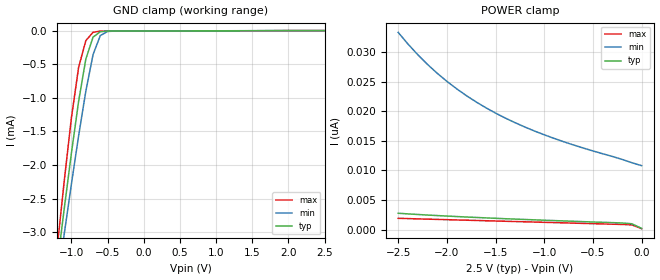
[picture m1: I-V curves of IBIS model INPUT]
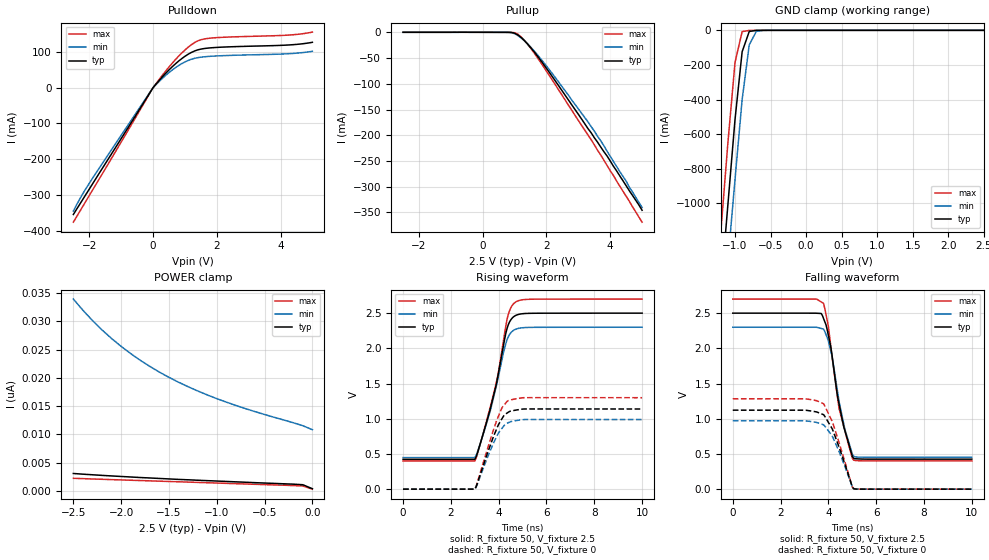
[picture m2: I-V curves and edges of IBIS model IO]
|   PERICOM SEMICONDUCTOR CORP
|   IBIS Model of PI4ULS3V204
|   Product Family: ULS
|   TSSOP-14 (L) Package
[IBIS Ver] 3.2
[Comment char] |_char
[File Name] pi4uls3v204_l_25v.ibs
[File Rev] 1.0
[Source] File originated at Pericom Semiconductor Corp.
[Date] 09/06/2017
[Disclaimer] (C) Copyright PERICOM Semiconductor Corporation
   All rights reserved
  Pericom Semiconductor Corporation hereby grants the user of
  this IBIS model a non-exclusive, nontransferable license to
  use this IBIS model under the following terms.
  This IBIS model is provided on an "AS IS" basis and Pericom
  makes absolutely no warranty with respect to the information
  contained herein. PERICOM DISCLAIMS AND CUSTOMER WAIVES ALL
  WARRANTIES, EXPRESSED OR IMPLIED, INCLUDING WARRANTIES OF
  MERCHANTABILITY OR FITNESS FOR A PARTICULAR PURPOSE. The
  entire risk as to quality and performance is with the customer.
  Accordingly, in no event shall the company be liable for any
  damages, whether in contract or tort, including any lost
  profits or other incidental, consequential, exemplary, or
  punitive damages arising out of the use or application of the
  IBIS model provided in this package. Further, Pericom reserves
  the right to make changes without notice to any product herein
  to improve reliability, function, or design. Pericom does not
  convey any license under patent rights or any other intellectual
  property rights, including those of third parties.
  The user is granted this license only to use the IBIS model
  and is not granted rights to sell, load, rent, lease or license
  the IBIS model in whole or in part, or in modified form to anyone
  other than user. User may modify the IBIS model to suit its specific
  application but rights to derivative works and such modifications
  shall belong to Pericom.
  Pericom is not obligated to provide maintenance or support
  for the licensed IBIS model.
  Contact Pericom at ATTN: APPLICATION ENGINEERING / IBIS MODELS
  1545 Barber Lane Milpitas, CA 95035 USA.
[Component] PI4ULS3V204
[Manufacturer] Pericom Semiconductor Corp.
[Package]
| variable   typ   min   max
R_pkg   0.04200   0.03995   0.04405
L_pkg   2.30669n   2.21200n   2.40138n
C_pkg   0.21108p   0.20715p   0.21500p
[Pin] signal_name  model_name   R_pin   L_pin   C_pin
1   VCCA   POWER   0.03604  2.91900n  0.20300p
2   A1   IO   0.03631  2.73467n  0.19100p
3   A2   IO   0.03658  2.55033n  0.17900p
4   A3   IO   0.03686  2.36600n  0.16700p
5   A4   IO   0.03658  2.55033n  0.17900p
6   NC   NC   0.03631  2.73467n  0.19100p
7   GND   GND   0.03604  2.91900n  0.20300p
8   EN   INPUT   0.03604  2.91900n  0.20300p
9   NC   NC   0.03631  2.73467n  0.19100p
10   B4   IO   0.03658  2.55033n  0.17900p
11   B3   IO   0.03686  2.36600n  0.16700p
12   B2   IO   0.03658  2.55033n  0.17900p
13   B1   IO   0.03631  2.73467n  0.19100p
14   VCCB   POWER   0.03604  2.91900n  0.20300p
| Models and submodels in the file (2): INPUT (Input), IO (I/O)
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[Model] INPUT
Model_type Input
Vinl = 750mV
Vinh = 1.75V
| variable   typ   min   max
C_comp   0.220pF   0.210pF   0.230pF
[Voltage Range]   2.5000V   2.3000V   2.7000V
[POWER Clamp Reference] 2.5000V   2.3000V   2.7000V
[GND Clamp Reference]   0.0000V   0.0000V   0.0000V
[Temperature Range]   25   85   -40
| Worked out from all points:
|   GND clamp passes 1 mA (typ) near -0.89 V on its own axis
[GND Clamp]
| Voltage   I(typ)   I(min)   I(max)
-2.5V     -15.24mA   -14.07mA   -17.39mA
-1.2V     -3.522mA   -3.797mA   -3.269mA
-1.1V     -2.66mA    -3.033mA   -2.25mA
-1V       -1.827mA   -2.286mA   -1.301mA
-900mV    -1.052mA   -1.566mA   -547.2uA
-800mV    -422.5uA   -898.9uA   -148.9uA
-700mV    -96.84uA   -355.4uA   -24.88uA
-600mV    -16.44uA   -73.79uA   -8.152uA
-500mV    -7.697uA   -13.25uA   -6.964uA
2.5V      368.1pA    666.4pA    17.74pA
[POWER Clamp]
| Voltage   I(typ)   I(min)   I(max)
-2.5V     2.782nA    33.28nA    1.93nA
-2.4V     2.672nA    31.33nA    1.882nA
-2.3V     2.573nA    29.54nA    1.829nA
-2.2V     2.48nA     27.9nA     1.789nA
-2V       2.305nA    25.03nA    1.698nA
-1.8V     2.143nA    22.62nA    1.61nA
-1.5V     1.929nA    19.67nA    1.474nA
-1.2V     1.732nA    17.33nA    1.342nA
-900mV    1.544nA    15.41nA    1.206nA
-700mV    1.429nA    14.3nA     1.114nA
-100mV    1.007nA    11.3nA     823.3pA
0V        230.9pA    10.81nA    182pA
[Model]   IO
Model_type I/O
Vinl=0.15
Vinh=2.2
Enable   Active-High
Vref =   2.5
Rref =   50
Cref =   15p
Vmeas =   1.25
| variable   typ   min   max
C_comp   3.670E-12   3.650E-12   3.690E-12
[Voltage Range]   2.5000V   2.3000V   2.7000V
[POWER Clamp Reference] 2.5000V   2.3000V   2.7000V
[GND Clamp Reference]   0.000E+00   0.000E+00   0.000E+00
[Pullup Reference]   2.5000V   2.3000V   2.7000V
[Pulldown Reference]   0.000E+00   0.000E+00   0.000E+00
[Temperature Range]   25   85   -40
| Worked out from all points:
|   slope of the pulldown table from 0 to 0.375 V, typ, clamps not added: 9.83 ohm
|   slope of the pullup table from 0 to 0.375 V, typ, clamps not added: 10.1 kohm
|   GND clamp passes 1 mA (typ) near -0.71 V on its own axis
|   rising waveform, R_fixture 50, V_fixture 2.5: 20-80 % time 827ps typ, 805ps min, 855ps max; typ from 0.426 V to 2.5 V
|   falling waveform, R_fixture 50, V_fixture 2.5: 20-80 % time 621ps typ, 592ps min, 640ps max; typ from 2.5 V to 0.428 V
|   rising waveform, R_fixture 50, V_fixture 0: 20-80 % time 735ps typ, 733ps min, 742ps max; typ from 0.002 V to 1.14 V
|   falling waveform, R_fixture 50, V_fixture 0: 20-80 % time 726ps typ, 715ps min, 738ps max; typ from 1.12 V to 0.002 V
[GND Clamp]
| Voltage   I(typ)   I(min)   I(max)
-2.5V     -7.893A    -7.937A    -7.872A
-1.2V     -1.497A    -1.804A    -1.164A
-1.1V     -1.005A    -1.332A    -648.2mA
-1V       -514.4mA   -860.5mA   -184.8mA
-900mV    -123.7mA   -400mA     -7.522mA
-800mV    -6.738mA   -83.76mA   -632.8uA
-700mV    -436.7uA   -5.934mA   -74.67uA
-500mV    -2.716uA   -28.54uA   -128.4nA
2.5V      406pA      12.07nA    40.1pA
[POWER Clamp]
| Voltage   I(typ)   I(min)   I(max)
-2.5V     3.102nA    33.93nA    2.247nA
-2.3V     2.873nA    30.14nA    2.127nA
-2.2V     2.764nA    28.48nA    2.076nA
-2V       2.572nA    25.57nA    1.964nA
-1.8V     2.386nA    23.11nA    1.854nA
-1.6V     2.221nA    21.02nA    1.742nA
-1.5V     2.138nA    20.09nA    1.684nA
-1.3V     1.985nA    18.44nA    1.578nA
-1V       1.766nA    16.33nA    1.41nA
-700mV    1.552nA    14.57nA    1.244nA
-100mV    1.113nA    11.55nA    895.1pA
0V        405.7pA    10.84nA    328.7pA
[Pullup]
| Voltage   I(typ)   I(min)   I(max)
-2.5V     20.34uA    13.34uA    33.35uA
800mV     -94.75uA   -159.8uA   -80.38uA
1V        -1.716mA   -2.726mA   -801.6uA
1.1V      -5.024mA   -6.194mA   -3.707mA
1.4V      -22.19mA   -22.02mA   -22.63mA
1.8V      -53.03mA   -49.94mA   -56.88mA
3.3V      -186.9mA   -173.8mA   -199.2mA
3.7V      -222.6mA   -210.5mA   -238mA
3.9V      -240.2mA   -230.9mA   -258.5mA
4.5V      -298mA     -289mA     -318.5mA
4.6V      -307.8mA   -301.1mA   -328.3mA
5V        -345.7mA   -340.3mA   -368.9mA
[Pulldown]
| Voltage   I(typ)   I(min)   I(max)
-2.5V     -354.2mA   -344.7mA   -375.7mA
-2.3V     -325.8mA   -311.1mA   -345.9mA
-2V       -283.2mA   -267.1mA   -301.3mA
0V        -247.5uA   -227.2uA   -267.8uA
300mV     30.71mA    26.4mA     35.35mA
600mV     58.1mA     49.09mA    67.93mA
900mV     80.97mA    67mA       96.49mA
1.1V      93.15mA    75.8mA     112.6mA
1.4V      105.4mA    83.64mA    130.4mA
1.7V      110.2mA    86.87mA    137.2mA
4.2V      118.8mA    94.49mA    146.5mA
5V        126.6mA    101.5mA    155.1mA
[Rising Waveform]
R_fixture = 50
V_fixture = 2.5
V_fixture_min = 2.3
V_fixture_max = 2.7
| Time   V(typ)   V(min)   V(max)
0s        425.8mV    450.1mV    402.5mV
3ns       425.8mV    450.1mV    402.5mV
3.45ns    900.6mV    887mV      916mV
3.9ns     1.486V     1.463V     1.513V
4.2ns     2.039V     1.94V      2.109V
4.35ns    2.281V     2.124V     2.413V
4.5ns     2.402V     2.219V     2.57V
4.7ns     2.465V     2.27V      2.655V
5.3ns     2.497V     2.298V     2.697V
10ns      2.5V       2.3V       2.7V
[Falling Waveform]
R_fixture = 50
V_fixture = 2.5
V_fixture_min = 2.3
V_fixture_max = 2.7
| Time   V(typ)   V(min)   V(max)
0s        2.5V       2.3V       2.7V
3.7ns     2.495V     2.283V     2.659V
3.8ns     2.422V     2.274V     2.638V
4ns       2.185V     2.105V     2.312V
4.15ns    1.909V     1.891V     1.892V
4.35ns    1.395V     1.46V      1.384V
4.45ns    1.207V     1.239V     1.143V
4.7ns     821.8mV    839mV      817.4mV
5.05ns    442.2mV    471.3mV    415.4mV
10ns      427.8mV    453.7mV    403.6mV
[Rising Waveform]
R_fixture = 50
V_fixture = 0
V_fixture_min = 0
V_fixture_max = 0
| Time   V(typ)   V(min)   V(max)
0s        1.954mV    2.014mV    1.89mV
3ns       1.954mV    2.013mV    1.89mV
3.1ns     75.4mV     64.74mV    88.23mV
3.5ns     482.5mV    425.3mV    539.3mV
3.9ns     845mV      737.2mV    960.1mV
4.15ns    1.009V     870.6mV    1.164V
4.25ns    1.06V      914.1mV    1.206V
4.4ns     1.093V     944.4mV    1.257V
5.05ns    1.14V      989.4mV    1.3V
10ns      1.14V      989.7mV    1.3V
[Falling Waveform]
R_fixture = 50
V_fixture = 0
V_fixture_min = 0
V_fixture_max = 0
| Time   V(typ)   V(min)   V(max)
0s        1.123V     972.3mV    1.285V
3ns       1.123V     972.2mV    1.285V
3.5ns     1.099V     949.6mV    1.259V
3.8ns     1.059V     915.4mV    1.214V
4.15ns    865.4mV    761.9mV    968.9mV
4.2ns     826mV      727.8mV    927.4mV
4.45ns    596mV      533.7mV    657.5mV
5ns       35.06mV    35.75mV    34.19mV
5.05ns    11.54mV    12.24mV    8.891mV
10ns      1.964mV    2.027mV    1.898mV
[Ramp]
| variable   typ   min   max
dV/dt_r   6.8270E-01/7.3200E-10  5.9270E-01/7.2268E-10  7.7900E-01/7.4241E-10
dV/dt_f   1.2433E+00/6.2057E-10  1.1078E+00/5.9230E-10  1.3778E+00/6.3973E-10
R_load = 50
